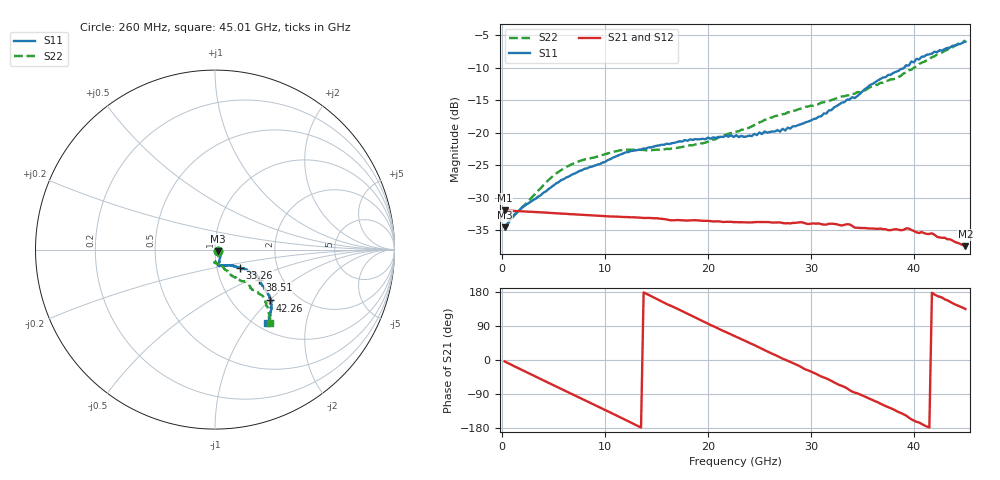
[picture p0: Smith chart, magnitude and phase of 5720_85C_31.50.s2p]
! Device:  ADRF5720
! Description: 0.5dB LSB GaAs MMIC 6-bit Digital Attenuator
! Frequency:  0.000009 -  40 GHz
! Ports:
!	RF1	= Port 1
!	RF2	= Port 2
! Vdd:  3.3 Volt
! Vss:  -3.3 Volt
! Control:  0/3.3 Volt
! State:  31.50 dB attenuation
! Data:  The device was measured using G-S-G Probes on a matrix board.
!  Data was collected using an calibrated 4 port network analyzer.
!  The reference plane for this measurement is at the launchers.
! Note:  Analog Devices supplies this data as a sample of measured data
!  for this product.  Your particular data for this product may vary.
!  Data was taken at 85 degrees C.
!  Analog Devices reserves the right to change this data at anytime.
# GHZ S DB R 45.0
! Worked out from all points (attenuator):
!   180 points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, 260 MHz to 45.01 GHz, reference 45 ohm
!   highest |S21| = -31.97 dB at 260 MHz (marker M1); lowest = -37.5 dB at 45.01 GHz (marker M2)
!   lowest |S11| = -34.6 dB at 260 MHz (marker M3), VSWR 1.04, Z = 46.6 - j0.718 ohm
!   |S11| at or under -10 dB: start of sweep to 39.07 GHz
!   |S22| runs from -34.8 to -5.8 dB; largest |S21 - S12| = 0.00021
!   S11 on the Smith chart (normalised r, x): 260 MHz: 1.03, -0.02; 33.26 GHz: 1.29, -0.27; 38.51 GHz: 1.53, -0.56; 42.26 GHz: 1.47, -1.01; 45.01 GHz: 1.12, -1.22
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0.26  -34.56 -24.3  -31.97 -3.7  -31.97 -3.7  -34.75 -26.4
1.76  -31.81 -4.5  -32.10 -23.9  -32.09 -23.8  -31.82 -20.6
4.76  -28.43 -39.0  -32.37 -63.3  -32.36 -63.3  -26.96 -65.7
6.26  -26.90 -47.8  -32.50 -82.9  -32.49 -82.8  -25.27 -75.1
7.76  -25.82 -54.8  -32.65 -102.4  -32.64 -102.3  -24.27 -81.6
11.51  -23.37 -69.4  -32.97 -151.6  -32.96 -151.4  -22.72 -92.1
15.26  -21.99 -76.0  -33.23 157.9  -33.22 158.0  -22.64 -89.8
19.51  -20.95 -77.3  -33.58 102.4  -33.57 102.6  -21.65 -76.6
22.76  -20.40 -72.2  -33.78 60.8  -33.77 61.0  -19.84 -67.4
23.51  -20.67 -71.7  -33.81 51.4  -33.80 51.6  -19.56 -65.3
25.51  -19.82 -64.4  -33.76 26.2  -33.74 26.4  -18.04 -63.5
27.01  -19.85 -59.1  -33.82 6.8  -33.80 7.0  -17.32 -60.0
30.26  -17.91 -45.2  -33.97 -33.4  -33.96 -33.2  -15.86 -58.7
33.26  -15.31 -36.2  -34.19 -71.0  -34.18 -70.8  -14.39 -53.9
37.76  -11.10 -32.0  -35.01 -127.1  -34.97 -126.7  -11.81 -46.1
38.51  -10.49 -34.0  -34.95 -137.4  -34.90 -137.0  -11.44 -46.0
39.51  -9.68 -36.9  -34.76 -151.9  -34.76 -151.7  -10.42 -46.8
40.26  -8.65 -38.9  -35.35 -163.2  -35.30 -162.5  -9.82 -45.6
41.76  -7.85 -41.6  -35.51 177.5  -35.47 177.6  -8.38 -44.3
42.26  -7.61 -42.9  -36.04 169.1  -36.04 169.7  -7.97 -45.2
43.51  -6.91 -45.5  -36.42 153.9  -36.38 154.1  -6.95 -48.7
45.01  -6.01 -54.3  -37.48 134.5  -37.43 134.8  -5.82 -53.3
